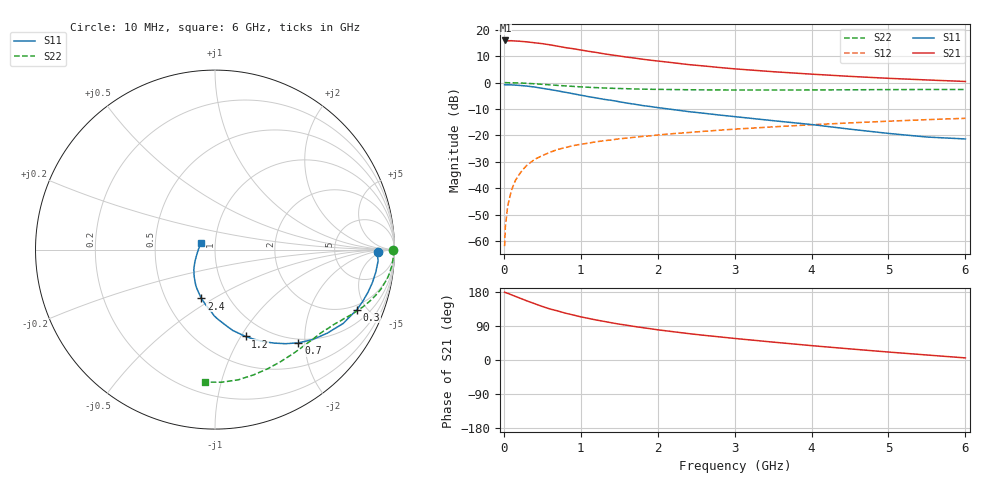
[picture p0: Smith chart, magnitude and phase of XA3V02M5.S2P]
! SIEMENS Discrete & RF Semiconductors
! BFY180
! Si NPN RF Bipolar Junction Transistor in MICRO-X
! VCE = 3 V  IC = 2.5 mA
! Common Emitter S-Parameters:  May  1997
# GHz  S  MA  R  50
!  f  S11  S21  S12  S22
! GHz  MAG  ANG  MAG  ANG  MAG  ANG  MAG  ANG
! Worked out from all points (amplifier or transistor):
!   36 points, 10 MHz to 6 GHz, reference 50 ohm
!   highest |S21| = 16.0 dB at 20 MHz (marker M1)
!   |S21| within 3 dB of that: start of sweep to 871.6 MHz
!   unconditionally stable (mu >= 1): 2.379 GHz to end of sweep
!   at 250 MHz: K = 0.16, MSG = 24.2 dB, |S12| = -32.8 dB
!   at 1.4 GHz: K = 0.77, MSG = 16.1 dB, |S12| = -21.7 dB
!   at 6 GHz: K = 1.07, MAG = 5.3 dB, |S12| = -13.5 dB
!   S11 on the Smith chart (normalised r, x): 10 MHz: 20, -3; 300 MHz: 1.69, -4.30; 700 MHz: 0.92, -1.87; 1.2 GHz: 0.80, -1.05; 2.4 GHz: 0.75, -0.44; 6 GHz: 0.85, +0.06
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0.01  0.9087 -0.9  6.215 178.9  0.0008 86.2  0.9935 -0.2
0.02  0.9049 -1.8  6.278 178.0  0.0019 83.5  0.9999 -0.8
0.05  0.911 -3.9  6.184 176.0  0.0046 86.3  0.9941 -1.7
0.1  0.9048 -7.9  6.206 172.0  0.0093 86.7  0.9927 -3.6
0.2  0.8849 -15.6  6.082 163.9  0.0183 80.7  0.9826 -7.2
0.3  0.8586 -22.9  5.906 156.0  0.0272 75.8  0.9671 -10.5
0.5  0.7795 -36.7  5.459 141.3  0.0415 68.7  0.9273 -16.3
0.6  0.7401 -42.6  5.19 134.6  0.048 65.0  0.9056 -18.8
0.7  0.6968 -48.2  4.886 129.5  0.0542 62.0  0.8853 -21.0
0.8  0.6556 -53.1  4.598 123.6  0.0589 60.0  0.8658 -23.0
0.9  0.6155 -57.8  4.385 118.9  0.064 57.3  0.8474 -24.9
1.1  0.5421 -66.8  3.916 109.8  0.0715 54.5  0.8154 -28.1
1.2  0.5131 -70.6  3.72 105.6  0.0758 52.8  0.8033 -29.7
1.4  0.4611 -77.6  3.344 98.2  0.0822 50.6  0.7808 -32.5
1.7  0.3897 -87.4  2.914 88.4  0.0923 48.0  0.7575 -36.5
2.2  0.3084 -100.2  2.376 74.7  0.1081 44.2  0.7376 -43.2
2.4  0.2824 -105.7  2.193 69.7  0.1133 43.1  0.7322 -45.6
3  0.2269 -118.2  1.821 56.9  0.1314 39.1  0.7248 -53.2
3.5  0.1902 -127.6  1.608 47.2  0.1452 36.1  0.7234 -59.6
4.5  0.1313 -148.7  1.312 29.3  0.1726 28.9  0.7302 -72.8
5.5  0.0932 -179.7  1.122 13.2  0.1988 21.3  0.7397 -87.0
6  0.0857 154.2  1.05 5.5  0.2107 17.1  0.7405 -94.1
